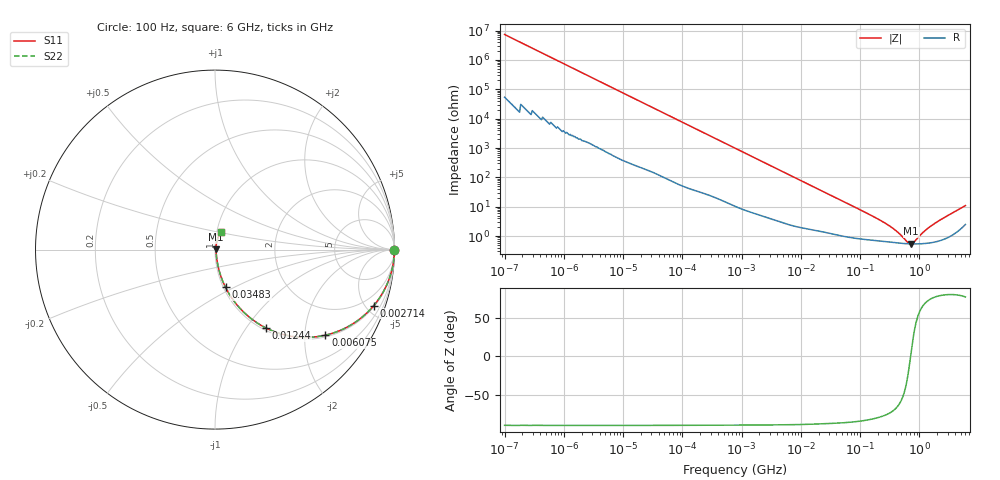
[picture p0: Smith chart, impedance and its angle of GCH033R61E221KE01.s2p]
!Murata Part Number: GCH033R61E221KE01
!These Parameters are Measured in Series Mode Connection
!Data Generated on Jun 19, 2026
!  o--ll--o
!Port1  Port2
!  o------o
!Operation Temp=25[degC], DC Bias Voltage=0[V]
!Freq. Start=100[Hz] Stop=6[GHz] 401[Steps]
# Hz S RI R 50
!Freq.(Hz) S11(Real) S11(Imag) S21(Real) S21(Imag) S12(Real) S12(Imag) S22(Real) S22(Imag)
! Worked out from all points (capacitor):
!   401 points, 100 Hz to 6 GHz, reference 50 ohm
!   read as one part in series: C = 217 pF near 109 Hz
!   lowest |Z| = 548 mohm at 731.5 MHz (marker M1)
!   series resonance near 713.5 MHz, so ESL is about 230 pH
!   S11 on the Smith chart (normalised r, x): 100 Hz: open; 2.714 MHz: 1.09, -5.65; 6.075 MHz: 1.05, -2.54; 12.44 MHz: 1.04, -1.25; 34.83 MHz: 1.02, -0.45; 6 GHz: 1.05, +0.21
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100  1 -1.36e-05  1e-07 1.36e-05  1e-07 1.36e-05  1 -1.36e-05
717  1 -9.7e-05  5e-07 9.7e-05  5e-07 9.7e-05  1 -9.7e-05
2008  1 -0.000271  1.4e-06 0.000271  1.4e-06 0.000271  1 -0.000271
40335  0.9999 -0.00539  6.37e-05 0.00539  6.37e-05 0.00539  0.9999 -0.00539
241822  0.9987 -0.032  0.00131 0.032  0.00131 0.032  0.9987 -0.032
774597  0.9887 -0.1007  0.0113 0.1007  0.0113 0.1007  0.9887 -0.1007
2713602  0.8848 -0.3117  0.1152 0.3117  0.1152 0.3117  0.8848 -0.3117
4060267  0.7779 -0.4072  0.2221 0.4072  0.2221 0.4072  0.7779 -0.4072
6075234  0.6148 -0.4769  0.3852 0.4769  0.3852 0.4769  0.6148 -0.4769
8692127  0.4431 -0.4852  0.5569 0.4852  0.5569 0.4852  0.4431 -0.4852
1.243624e7  0.2857 -0.4377  0.7143 0.4377  0.7143 0.4377  0.2857 -0.4377
1.555665e7  0.2077 -0.3896  0.7923 0.3896  0.7923 0.3896  0.2077 -0.3896
3.482834e7  0.0586 -0.2103  0.9414 0.2103  0.9414 0.2103  0.0586 -0.2103
8.918374e7  0.0158 -0.0865  0.9842 0.0865  0.9842 0.0865  0.0158 -0.0865
3.124326e8  0.00666 -0.0213  0.9933 0.0213  0.9933 0.0213  0.00666 -0.0213
4.274388e8  0.00596 -0.0125  0.994 0.0125  0.994 0.0125  0.00596 -0.0125
6.395615e8  0.00547 -0.0026  0.9945 0.0026  0.9945 0.0026  0.00547 -0.0026
7.31507e8  0.00542 0.000599  0.9946 -0.000599  0.9946 -0.000599  0.00542 0.000599
8.000355e8  0.00541 0.00274  0.9946 -0.00274  0.9946 -0.00274  0.00541 0.00274
1.197065e9  0.00572 0.013  0.9943 -0.013  0.9943 -0.013  0.00572 0.013
1.712697e9  0.00667 0.0239  0.9933 -0.0239  0.9933 -0.0239  0.00667 0.0239
6e9  0.0347 0.1002  0.9653 -0.1002  0.9653 -0.1002  0.0347 0.1002
